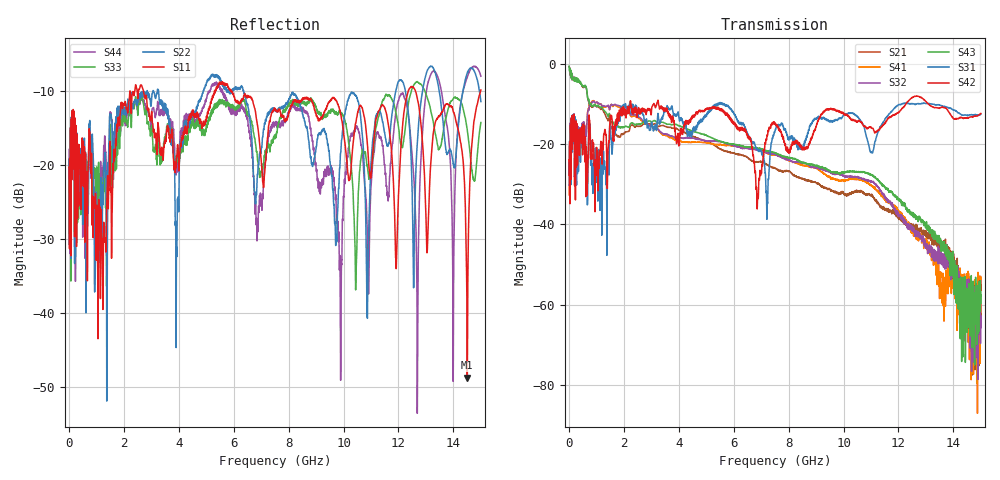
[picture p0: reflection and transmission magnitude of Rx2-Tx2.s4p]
! FILE: N:\QM 2007\Prüfprotokolle\Highspeed\Konfektionierte Ltg\L45593-D106\D30\8216\0002  kpl\IL  mit Chris Boards\Rx2-Tx2.s4p
# MHz S DB R 50.00
! FREQ  S11  S12  S13  S14
!  S21  S22  S23  S24
!  S31  S32  S33  S34
!  S41  S42  S43  S44
!  DB  ANG  DB  ANG  DB  ANG  DB  ANG
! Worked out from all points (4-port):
!   2999 points, 10 MHz to 15 GHz, reference 50 ohm
!   strongest paths, dB at 10 MHz, 3.755 GHz, 7.505 GHz, 11.26 GHz, 15 GHz:
!     S42: -23.8, -13.1, -14.8, -16.4, -12.3
!     S31: -24.6, -10.5, -16.6, -16.8, -12.5
!     S43: -0.5, -15.2, -22.1, -29.0, -59.7
!     S32: -30.3, -18.0, -22.5, -30.7, -65.7
!     S41: -32.6, -18.5, -22.6, -31.9, -55.2
!     S21: -0.6, -16.0, -26.0, -34.8, -63.3
!   lowest |S11| = -48.8 dB at 14.51 GHz (marker M1), VSWR 1.01, Z = 50.1 + j0.336 ohm
!   |S11| at or under -10 dB: 2.716 GHz to 5.329 GHz (2.613 GHz wide, 65 % of centre); 5.925 GHz to 12.36 GHz (6.433 GHz wide, 70.4 % of centre); 12.62 GHz to 14.99 GHz (2.379 GHz wide, 17.2 % of centre)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
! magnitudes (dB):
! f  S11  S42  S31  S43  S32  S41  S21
! 10 MHz  -20.3  -23.8  -24.6  -0.5  -30.3  -32.6  -0.6
! 8.49 GHz  -11.2  -21.4  -21.3  -24.6  -24.6  -25.2  -28.6
! 9.875 GHz  -12.7  -11.9  -13.5  -27.3  -27.7  -29.1  -32.2
! 12.13 GHz  -15.3  -11.0  -10.0  -34.4  -38.0  -38.3  -38.5
! 12.69 GHz  -11.0  -8.0  -9.9  -38.3  -43.0  -43.8  -41.3
! 14.51 GHz  -48.8  -13.5  -12.8  -66.9  -62.7  -66.4  -57.2
! 15 GHz  -9.9  -12.3  -12.5  -59.7  -65.7  -55.2  -63.3
